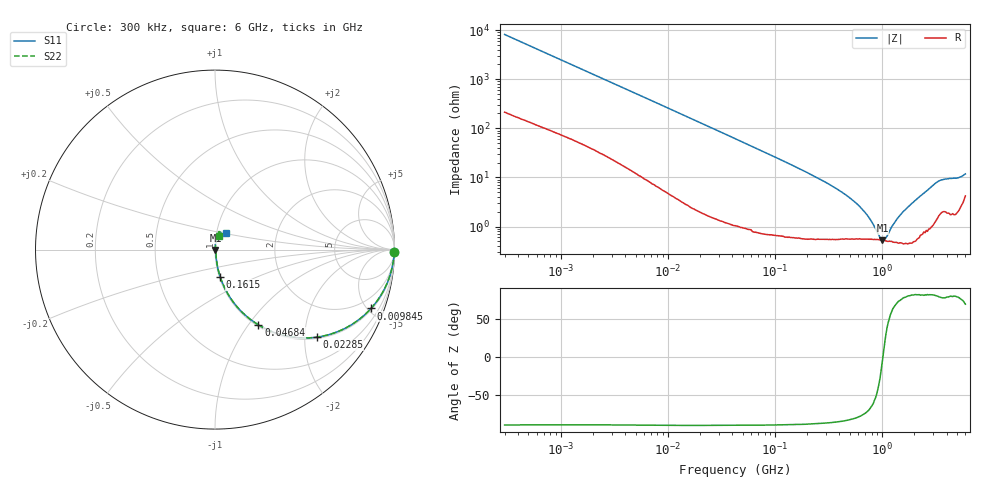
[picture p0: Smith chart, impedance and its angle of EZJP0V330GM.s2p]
!*** S-Parameter ***
!Copyright  (C)  Panasonic Corporation
!Multilaryer Varistors, Chip Type  Port assignments : Series-thru
!  1  o---GGG---o  2
!Parts No. : EZJP0V330GM  GND o---------o GND
# HZ S RI R 50
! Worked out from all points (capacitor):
!   401 points, 300 kHz to 6 GHz, reference 50 ohm
!   read as one part in series: C = 65.1 pF near 315.2 kHz
!   lowest |Z| = 527 mohm at 1.009 GHz (marker M1)
!   series resonance near 1.019 GHz, so ESL is about 380 pH
!   S11 on the Smith chart (normalised r, x): 300 kHz: open; 9.845 MHz: 1.10, -5.27; 22.85 MHz: 1.04, -2.29; 46.84 MHz: 1.02, -1.12; 161.5 MHz: 1.01, -0.32; 6 GHz: 1.11, +0.21
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300000  0.9995 -0.0128  0.000478 0.0123  0.000484 0.0123  0.9993 -0.0126
1575955  0.9939 -0.062  0.00576 0.0622  0.00576 0.0622  0.9938 -0.0622
8278775  0.9029 -0.2867  0.0973 0.2867  0.0973 0.2867  0.9025 -0.2868
9845415  0.8697 -0.3276  0.1303 0.3276  0.1303 0.3277  0.8693 -0.3275
2.284659e7  0.5663 -0.488  0.4337 0.4884  0.4338 0.4884  0.566 -0.4879
4.348989e7  0.2697 -0.4353  0.7299 0.4355  0.7299 0.4358  0.2692 -0.4348
4.684315e7  0.2419 -0.4194  0.7575 0.4199  0.7576 0.4201  0.2416 -0.4191
1.615379e8  0.0293 -0.1523  0.9698 0.1528  0.9698 0.1529  0.0292 -0.1514
2.228734e8  0.0169 -0.1087  0.9817 0.1091  0.9818 0.1091  0.0168 -0.1075
4.242534e8  0.00701 -0.0486  0.9911 0.0496  0.9913 0.0497  0.0071 -0.0465
6.462772e8  0.00461 -0.0226  0.9928 0.0232  0.993 0.0231  0.00519 -0.0196
8.485886e8  0.00322 -0.00958  0.9927 0.00867  0.9929 0.00848  0.00442 -0.00613
9.369307e8  0.00289 -0.00541  0.9929 0.00397  0.9929 0.0036  0.00427 -0.0019
1.009172e9  0.00246 -0.00239  0.9926 0.000274  0.9929 0.000122  0.00394 0.00114
1.086984e9  0.00211 0.000615  0.9926 -0.00327  0.9929 -0.00357  0.00382 0.00402
1.170796e9  0.00175 0.00327  0.9923 -0.00705  0.9928 -0.00726  0.00345 0.00661
1.292679e9  0.00112 0.00705  0.9922 -0.012  0.9925 -0.0123  0.00304 0.0101
1.499708e9  0.000839 0.0129  0.9918 -0.0197  0.992 -0.0201  0.00264 0.015
3.151982e9  0.0208 0.0811  0.9849 -0.0656  0.9818 -0.066  0.0175 0.0785
4.13868e9  0.031 0.0956  0.9756 -0.0792  0.9732 -0.0751  0.0237 0.1003
5.301363e9  0.0205 0.0682  0.9496 -0.1154  0.9534 -0.114  0.00782 0.0734
6e9  0.0617 0.0926  0.937 -0.1187  0.939 -0.111  0.0204 0.0778
